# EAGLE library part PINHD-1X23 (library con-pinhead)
PIN HEADER
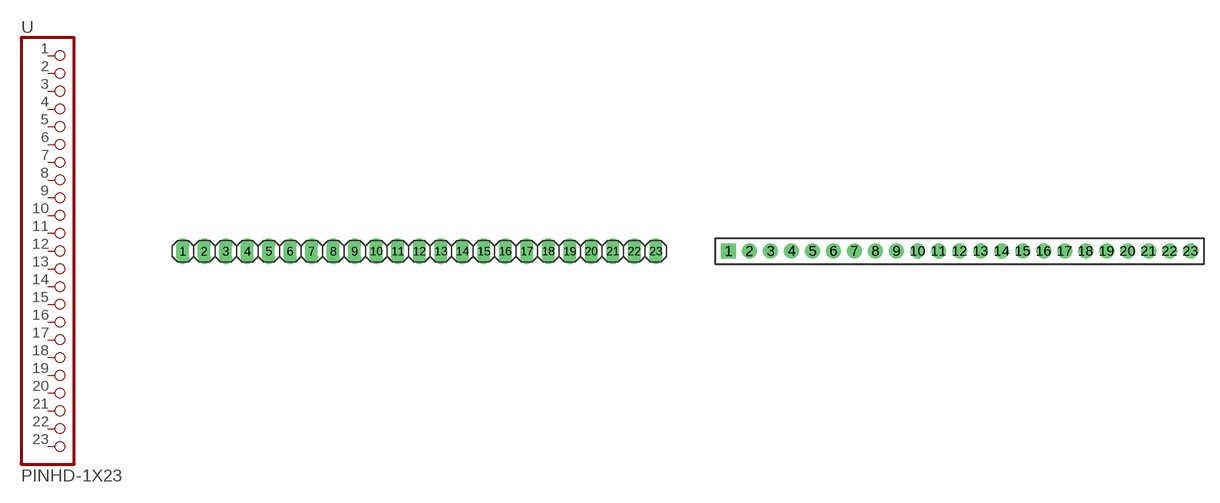
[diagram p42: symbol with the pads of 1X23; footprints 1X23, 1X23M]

Designator prefix -

## PINHD-1X23_2.54  [1X23]
1  1  pas
2  2  pas
3  3  pas
4  4  pas
5  5  pas
6  6  pas
7  7  pas
8  8  pas
9  9  pas
10  10  pas
11  11  pas
12  12  pas
13  13  pas
14  14  pas
15  15  pas
16  16  pas
17  17  pas
18  18  pas
19  19  pas
20  20  pas
21  21  pas
22  22  pas
23  23  pas

## PINHD-1X23_2.00  [1X23M]
Pads as for 1X23

## PINHD-1X23_2.54-90°  [1X23/90]
Pads as for 1X23

## PINHD-1X23_2.54-SMD  [1X23SMD]
Pads as for 1X23

## PINHD-1X23_2.54-SMD-90°  [1X23SMD/90]
Pads as for 1X23

## Footprint 1X23 (pad centres in mm)
PIN HEADER - 2.54
drill 1.016 long: 1 -26.67,0; 2 -24.13,0; 3 -21.59,0; 4 -19.05,0; 5 -16.51,0; 6 -13.97,0; 7 -11.43,0; 8 -8.89,0; 9 -6.35,0; 10 -3.81,0; 11 -1.27,0; 12 1.27,0; 13 3.81,0; 14 6.35,0; 15 8.89,0; 16 11.43,0; 17 13.97,0; 18 16.51,0; 19 19.05,0; 20 21.59,0; 21 24.13,0; 22 26.67,0; 23 29.21,0

## Footprint 1X23M (pad centres in mm)
PIN HEADER - 2
drill 0.914 square: 1 -21,0
drill 0.914: 2 -19,0; 3 -17,0; 4 -15,0; 5 -13,0; 6 -11,0; 7 -9,0; 8 -7,0; 9 -5,0; 10 -3,0; 11 -1,0; 12 1,0; 13 3,0; 14 5,0; 15 7,0; 16 9,0; 17 11,0; 18 13,0; 19 15,0; 20 17,0; 21 19,0; 22 21,0; 23 23,0

## Footprint 1X23/90 (pad centres in mm)
PIN HEADER - 2.54 90°
drill 1.016 long: 1 -24.13,-3.81; 2 -21.59,-3.81; 3 -19.05,-3.81; 4 -16.51,-3.81; 5 -13.97,-3.81; 6 -11.43,-3.81; 7 -8.89,-3.81; 8 -6.35,-3.81; 9 -3.81,-3.81; 10 -1.27,-3.81; 11 1.27,-3.81; 12 3.81,-3.81; 13 6.35,-3.81; 14 8.89,-3.81; 15 11.43,-3.81; 16 13.97,-3.81; 17 16.51,-3.81; 18 19.05,-3.81; 19 21.59,-3.81; 20 24.13,-3.81; 21 26.67,-3.81; 22 29.21,-3.81; 23 31.75,-3.81

## Footprint 1X23SMD (pad centres in mm)
PIN HEADER - 2.54 SMD
smd 1.016 x 3.302: 1 -1.27,1.27; 2 1.27,-1.27; 3 3.81,1.27; 4 6.35,-1.27; 5 8.89,1.27; 6 11.43,-1.27; 7 13.97,1.27; 8 16.51,-1.27; 9 19.05,1.27; 10 21.59,-1.27; 11 24.13,1.27; 12 26.67,-1.27; 13 29.21,1.27; 14 31.75,-1.27; 15 34.29,1.27; 16 36.83,-1.27; 17 39.37,1.27; 18 41.91,-1.27; 19 44.45,1.27; 20 46.99,-1.27; 21 49.53,1.27; 22 52.07,-1.27; 23 54.61,1.27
